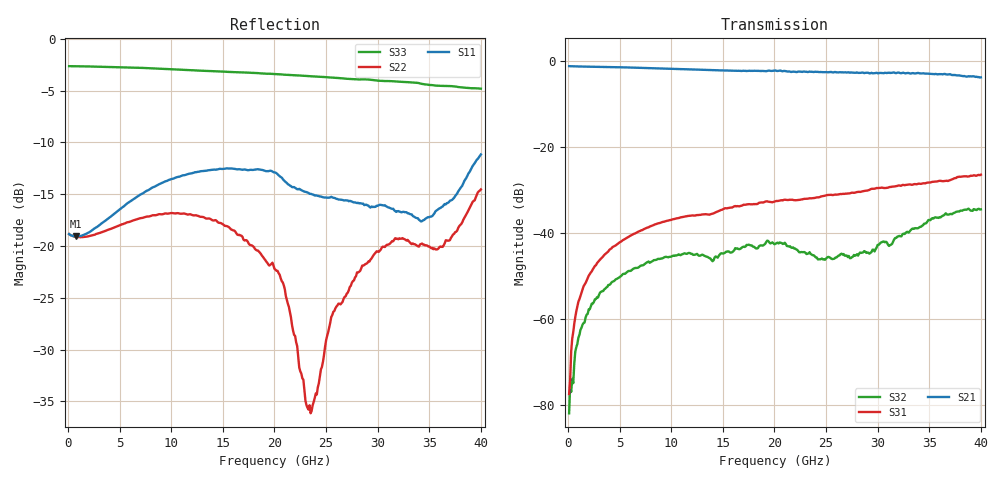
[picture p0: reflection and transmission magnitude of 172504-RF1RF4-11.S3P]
!  3-Port S-parameters saved by WinCal
! VAR MeasName=S-Parameters (CALIBRATED_DATA) read from VNA (N5245A)
! VAR MeasDate=2017-3-15 11:11:56
! VAR NAME=172504-RF1RF4-11
! VAR FILENAME=172504-RF1RF4-11.S3P
! VAR DATE=2017-3-15 11:11:56
! VAR PHYS_PORTS=1,2,3
# Hz S DB R 50
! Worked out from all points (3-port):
!   400 points, 100 MHz to 40 GHz, reference 50 ohm
!   strongest paths, dB at 100 MHz, 10.1 GHz, 20.1 GHz, 30.1 GHz, 40 GHz:
!     S21: -1.1, -1.7, -2.1, -2.7, -3.7
!     S31: -77.4, -36.7, -32.5, -29.4, -26.3
!     S32: -81.8, -45.3, -42.4, -42.7, -34.4
!   lowest |S11| = -19.1 dB at 800 MHz (marker M1), VSWR 1.25, Z = 61.9 - j3.69 ohm
!   |S11| at or under -10 dB: start of sweep to end of sweep
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1e8  -18.85 -2.6  -1.10 -0.7  -76.00 54.8
     -1.10 -0.7  -18.85 -2.4  -82.85 -164.7
     -77.37 113.0  -81.85 -172.5  -2.64 179.8
4e8  -19.02 -8.4  -1.13 -2.7  -65.31 101.9
     -1.13 -2.7  -19.01 -7.3  -76.79 103.0
     -64.50 104.4  -73.83 125.4  -2.64 179.1
8e8  -19.07 -15.3  -1.16 -5.1  -58.05 92.8
     -1.16 -5.1  -19.13 -13.1  -66.34 100.4
     -58.07 92.6  -66.46 102.7  -2.64 178.3
2.3e9  -18.50 -38.1  -1.23 -14.0  -48.59 81.4
       -1.23 -14.0  -18.99 -33.4  -56.66 81.0
       -48.79 81.6  -56.33 81.4  -2.67 175.2
5.8e9  -15.84 -77.6  -1.38 -34.4  -40.85 61.5
       -1.40 -34.4  -17.71 -74.7  -48.84 51.0
       -40.88 61.8  -48.82 50.9  -2.76 168.1
2.01e10  -12.91 -157.2  -2.17 -114.8  -32.21 -1.9
         -2.10 -114.8  -22.30 173.5  -41.93 -41.0
         -32.50 -1.3  -42.38 -42.7  -3.39 138.3
2.35e10  -14.96 -163.2  -2.46 -134.0  -31.78 -17.3
         -2.39 -134.0  -36.16 58.5  -44.54 -69.2
         -31.83 -15.4  -44.76 -66.8  -3.61 130.1
2.8e10  -15.86 -173.8  -2.69 -161.1  -30.33 -36.2
        -2.55 -161.1  -22.55 -44.1  -44.92 -60.2
        -30.38 -34.6  -44.84 -58.1  -3.91 118.8
3.43e10  -17.60 122.5  -2.86 157.9  -28.33 -72.6
         -2.77 158.2  -19.76 -64.6  -38.76 -84.2
         -28.40 -69.9  -38.24 -79.9  -4.35 99.9
4e10  -11.16 31.5  -3.77 117.5  -26.10 -109.4
      -3.71 115.5  -14.54 -41.8  -34.37 -139.4
      -26.34 -107.8  -34.42 -141.1  -4.81 82.8
